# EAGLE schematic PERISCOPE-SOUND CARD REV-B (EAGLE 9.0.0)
This Set of Many Schematics Is what comprises the Revision-B PCB, of my eden project "PERISCOPE". (OBJECT BOARD ONLY)

## Sheet 1 of 3: SOUND
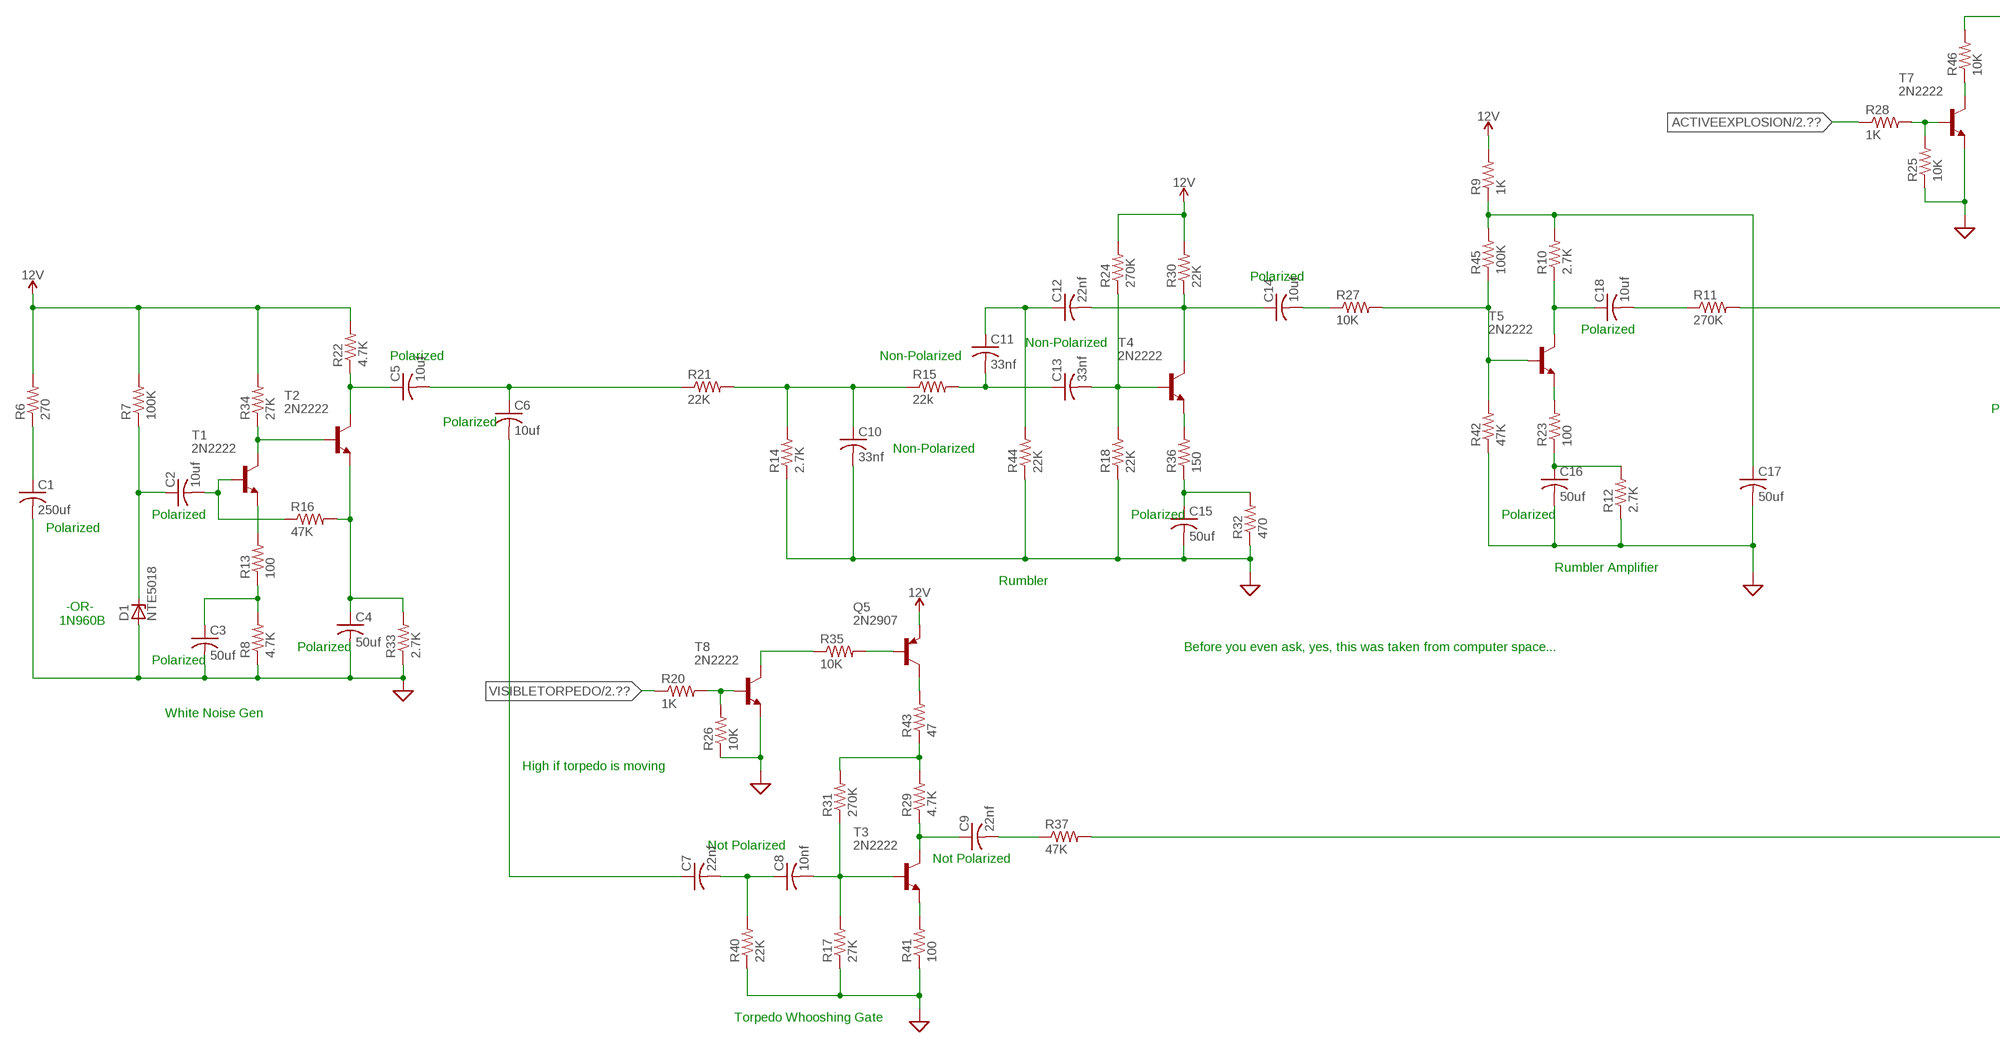
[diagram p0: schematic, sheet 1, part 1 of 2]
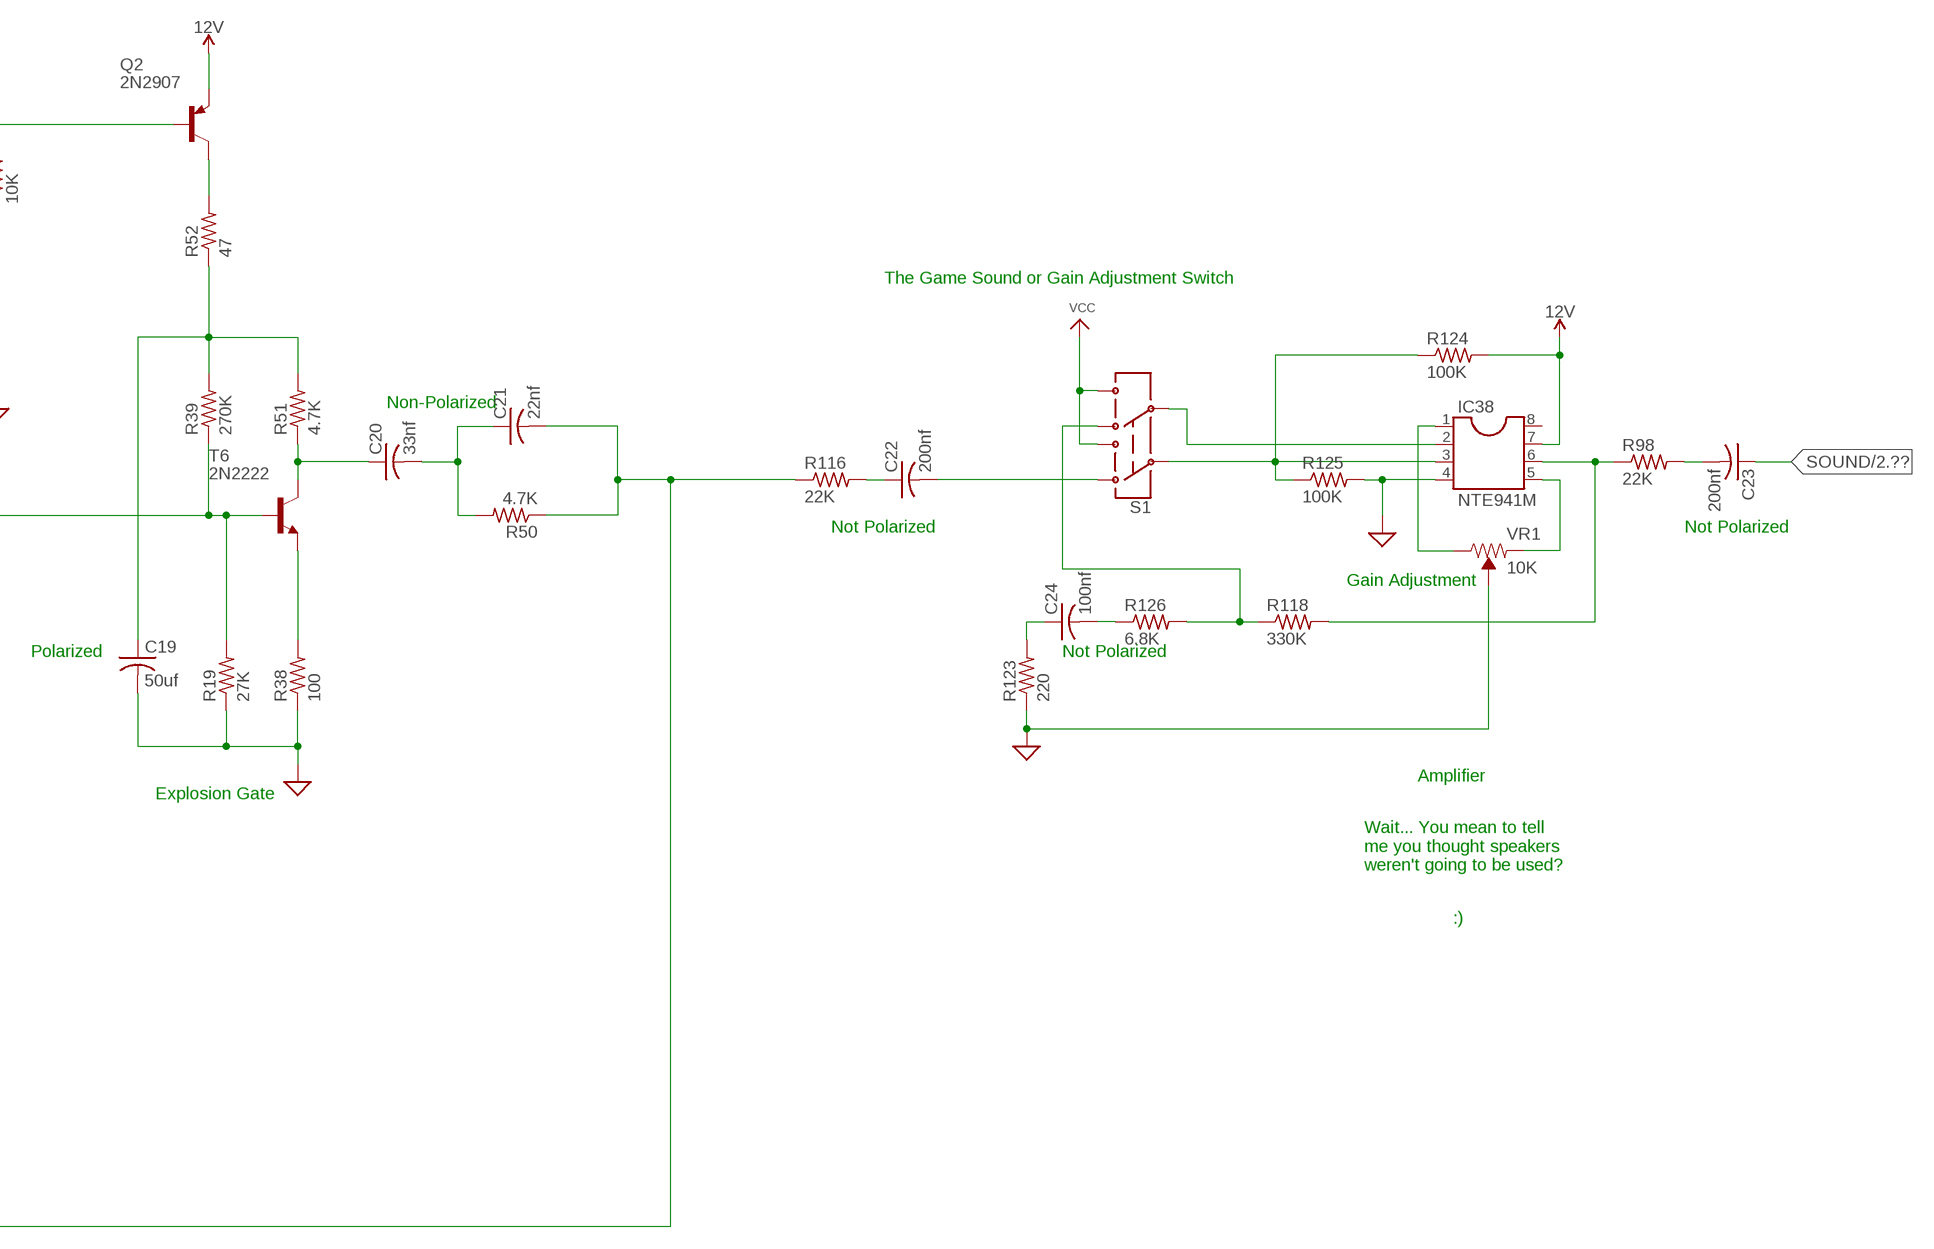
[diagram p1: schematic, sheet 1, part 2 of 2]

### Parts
C1  250uf  C-US025-050X050  [C025-050X050]
C2  10uf  C-US025-050X050  [C025-050X050]
C3  50uf  C-US025-050X050  [C025-050X050]
C4  50uf  C-US025-050X050  [C025-050X050]
C5  10uf  C-US025-050X050  [C025-050X050]
C6  10uf  C-US025-050X050  [C025-050X050]
C7  22nf  C-US025-050X050  [C025-050X050]
C8  10nf  C-US025-050X050  [C025-050X050]
C9  22nf  C-US025-050X050  [C025-050X050]
C10  33nf  C-US025-050X050  [C025-050X050]
C11  33nf  C-US025-050X050  [C025-050X050]
C12  22nf  C-US025-050X050  [C025-050X050]
C13  33nf  C-US025-050X050  [C025-050X050]
C14  10uf  C-US025-050X050  [C025-050X050]
C15  50uf  C-US025-050X050  [C025-050X050]
C16  50uf  C-US025-050X050  [C025-050X050]
C17  50uf  C-US025-050X050  [C025-050X050]
C18  10uf  C-US025-050X050  [C025-050X050]
C19  50uf  C-US025-050X050  [C025-050X050]
C20  33nf  C-US025-050X050  [C025-050X050]
C21  22nf  C-US025-050X050  [C025-050X050]
C22  200nf  C-US050-025X075  [C050-025X075]
C23  200nf  C-US050-025X075  [C050-025X075]
C24  100nf  C-US050-025X075  [C050-025X075]
D1  NTE5018  1N4728  [DO41Z10]
IC38  NTE941M  DIL8S  [SOCKET-08]
Q2  2N2907  [TO92-EBC-OVAL]
Q5  2N2907  [TO92-EBC-OVAL]
R6  270  R-US_0207/10  [0207/10]
R7  100K  R-US_0207/10  [0207/10]
R8  4.7K  R-US_0207/10  [0207/10]
R9  1K  R-US_0207/10  [0207/10]
R10  2.7K  R-US_0207/10  [0207/10]
R11  270K  R-US_0207/10  [0207/10]
R12  2.7K  R-US_0207/10  [0207/10]
R13  100  R-US_0207/10  [0207/10]
R14  2.7K  R-US_0207/10  [0207/10]
R15  22k  R-US_0207/10  [0207/10]
R16  47K  R-US_0207/10  [0207/10]
R17  27K  R-US_0207/10  [0207/10]
R18  22K  R-US_0207/10  [0207/10]
R19  27K  R-US_0207/10  [0207/10]
R20  1K  R-US_0207/10  [0207/10]
R21  22K  R-US_0207/10  [0207/10]
R22  4.7K  R-US_0207/10  [0207/10]
R23  100  R-US_0207/10  [0207/10]
R24  270K  R-US_0207/10  [0207/10]
R25  10K  R-US_0207/10  [0207/10]
R26  10K  R-US_0207/10  [0207/10]
R27  10K  R-US_0207/10  [0207/10]
R28  1K  R-US_0207/10  [0207/10]
R29  4.7K  R-US_0207/10  [0207/10]
R30  22K  R-US_0207/10  [0207/10]
R31  270K  R-US_0207/10  [0207/10]
R32  470  R-US_0207/10  [0207/10]
R33  2.7K  R-US_0207/10  [0207/10]
R34  27K  R-US_0207/10  [0207/10]
R35  10K  R-US_0207/10  [0207/10]
R36  150  R-US_0207/10  [0207/10]
R37  47K  R-US_0207/10  [0207/10]
R38  100  R-US_0207/10  [0207/10]
R39  270K  R-US_0207/10  [0207/10]
R40  22K  R-US_0207/10  [0207/10]
R41  100  R-US_0207/10  [0207/10]
R42  47K  R-US_0207/10  [0207/10]
R43  47  R-US_0207/10  [0207/10]
R44  22K  R-US_0207/10  [0207/10]
R45  100K  R-US_0207/10  [0207/10]
R46  10K  R-US_0207/10  [0207/10]
R50  4.7K  R-US_0207/10  [0207/10]
R51  4.7K  R-US_0207/10  [0207/10]
R52  47  R-US_0207/10  [0207/10]
R98  22K  R-US_0207/10  [0207/10]
R116  22K  R-US_0207/10  [0207/10]
R118  330K  R-US_0207/10  [0207/10]
R123  220  R-US_0207/10  [0207/10]
R124  100K  R-US_0207/10  [0207/10]
R125  100K  R-US_0207/10  [0207/10]
R126  6.8K  R-US_0207/10  [0207/10]
S1  SWITCH-DPDTPTH1  [MS]
T1  2N2222  [TO92-EBC-OVAL]
T2  2N2222  [TO92-EBC-OVAL]
T3  2N2222  [TO92-EBC-OVAL]
T4  2N2222  [TO92-EBC-OVAL]
T5  2N2222  [TO92-EBC-OVAL]
T6  2N2222  [TO92-EBC-OVAL]
T7  2N2222  [TO92-EBC-OVAL]
T8  2N2222  [TO92-EBC-OVAL]
VR1  10K  TRIMPOT-PTH-10MM-KNOB-1/2W-10%  [TRIMPOT-PTH-3386U]

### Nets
12V: IC38.7 Q2.E Q5.E R6.2 R7.2 R9.2 R22.2 R24.2 R30.2 R34.2 R124.2 ; also sheet 2
ACTIVEEXPLOSION: R28.1 ; also sheet 2,3
GND: C1.2 C3.2 C4.2 C10.2 C15.2 C16.2 C17.2 C19.2 D1.A IC38.4 R8.1 R12.1 R14.1 R17.1 R18.1 R19.1 R25.1 R26.1 R32.1 R33.1 R38.1 R40.1 R41.1 R42.1 R44.1 R123.1 R125.2 T7.E T8.E VR1.2(WIPER) ; supply symbol labelled SUP ; also sheet 2
N$1: C21.2 R37.2 R50.1 R116.1
N$3: R13.2 T1.E
N$4: C1.1 R6.1
N$5: C2.1 D1.C R7.1
N$6: C3.1 R8.2 R13.1
N$7: C9.2 R37.1
N$8: C2.2 R16.1 T1.B
N$10: R34.1 T1.C T2.B
N$11: C4.1 R16.2 R33.2 T2.E
N$12: C10.1 R14.2 R15.1 R21.2
N$13: C5.1 R22.1 T2.C
N$14: C5.2 C6.1 R21.1
N$15: C6.2 C7.1
N$16: C7.2 C8.1 R40.2
N$17: C11.2 C13.1 R15.2
N$18: C8.2 R17.2 R31.1 T3.B
N$19: R29.2 R31.2 R43.1
N$20: C9.1 R29.1 T3.C
N$21: R41.2 T3.E
N$22: Q5.C R43.2
N$23: Q5.B R35.2
N$24: R35.1 T8.C
N$25: R20.2 R26.2 T8.B
N$26: C11.1 C12.1 R44.2
N$27: C12.2 C14.1 R30.1 T4.C
N$28: C13.2 R18.2 R24.1 T4.B
N$29: R36.2 T4.E
N$30: C15.1 R32.2 R36.1
N$31: R27.2 R42.2 R45.1 T5.B
N$32: C14.2 R27.1
N$33: Q2.B R46.2
N$34: C16.1 R12.2 R23.1
N$35: R23.2 T5.E
N$36: C18.1 R10.1 T5.C
N$37: C17.1 R9.1 R10.2 R45.2
N$38: C18.2 R11.1
N$39: R11.2 R19.2 R39.1 T6.B
N$40: R25.2 R28.2 T7.B
N$42: R46.1 T7.C
N$43: Q2.C R52.2
N$44: C20.2 C21.1 R50.2
N$45: C19.1 R39.2 R51.2 R52.1
N$46: C20.1 R51.1 T6.C
N$47: R38.2 T6.E
N$117: IC38.2 S1.5
N$118: IC38.5 VR1.1(CCW)
N$169: R118.1 R126.2 S1.4
N$178: C22.1 R116.2
N$180: C22.2 S1.1
N$181: C23.2 R98.2
N$182: IC38.1 VR1.3(CW)
N$184: IC38.6 R98.1 R118.2
N$188: IC38.3 R124.1 R125.1 S1.2
N$193: C24.1 R123.2
N$194: C24.2 R126.1
SOUND: C23.1 ; also sheet 2,3
VCC: S1.3 S1.6
VISIBLETORPEDO: R20.1 ; also sheet 2,3
Unconnected: IC38.8

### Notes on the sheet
- The Game Sound or Gain Adjustment Switch
- Non-Polarized
- Polarized
- Not Polarized | Not Polarized
- Polarized
- Non-Polarized
- Polarized | Non-Polarized | Gain Adjustment
- Polarized | Not Polarized
- Polarized
- Non-Polarized
- Amplifier
- Polarized | Polarized | Polarized | Explosion Gate
- Polarized
- Rumbler Amplifier
- Wait... You mean to tell
  me you thought speakers
  weren't going to be used?
- Rumbler
- :)
- -OR-
  1N960B
- Polarized | Before you even ask, yes, this was taken from computer space...
- Polarized
- White Noise Gen
- High if torpedo is moving
- Not Polarized
- Not Polarized
- Torpedo Whooshing Gate

## Sheet 2 of 3: Signal Connectors
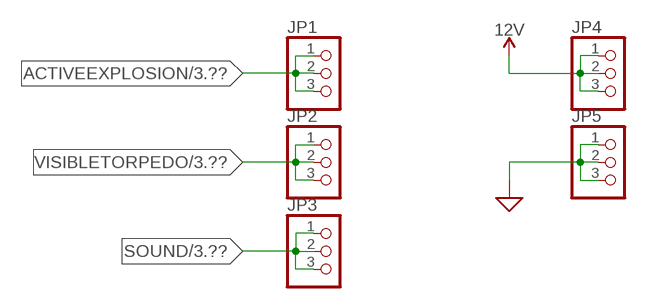
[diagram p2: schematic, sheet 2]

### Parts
JP1  PINHD-1X3  [1X03]
JP2  PINHD-1X3  [1X03]
JP3  PINHD-1X3  [1X03]
JP4  PINHD-1X3  [1X03]
JP5  PINHD-1X3  [1X03]

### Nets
12V: JP4.1 JP4.2 JP4.3 ; also sheet 1
ACTIVEEXPLOSION: JP1.1 JP1.2 JP1.3 ; also sheet 1,3
GND: JP5.1 JP5.2 JP5.3 ; supply symbol labelled SUP ; also sheet 1
SOUND: JP3.1 JP3.2 JP3.3 ; also sheet 1,3
VISIBLETORPEDO: JP2.1 JP2.2 JP2.3 ; also sheet 1,3

## Sheet 3 of 3: Alt. Sound
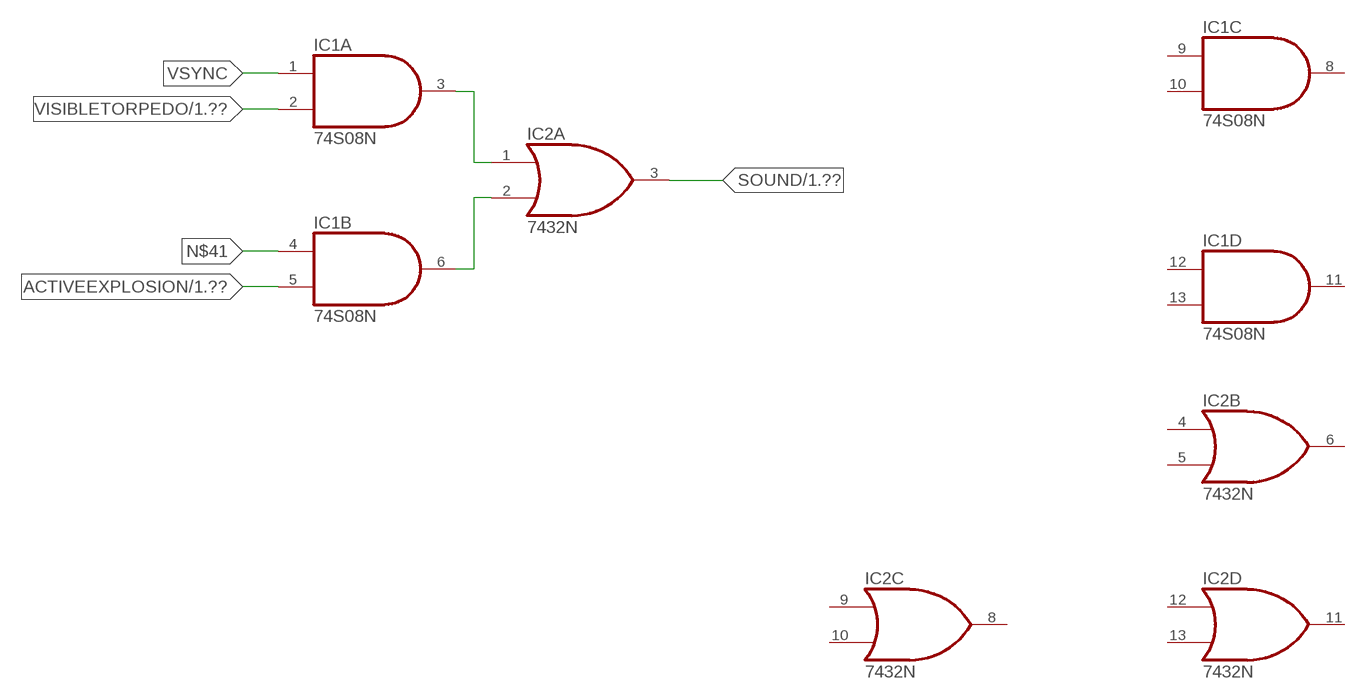
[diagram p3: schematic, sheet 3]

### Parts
IC1  74S08N  [DIL14]
IC2  7432N  [DIL14]

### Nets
ACTIVEEXPLOSION: IC1.5(B:I1) ; also sheet 1,2
N$2: IC1.3(A:O) IC2.1(A:I0)
N$9: IC1.6(B:O) IC2.2(A:I1)
N$41: IC1.4(B:I0)
SOUND: IC2.3(A:O) ; also sheet 1,2
VISIBLETORPEDO: IC1.2(A:I1) ; also sheet 1,2
VSYNC: IC1.1(A:I0)
Unconnected: IC1.8(C:O) IC1.9(C:I0) IC1.10(C:I1) IC1.11(D:O) IC1.12(D:I0) IC1.13(D:I1) IC2.4(B:I0) IC2.5(B:I1) IC2.6(B:O) IC2.8(C:O) IC2.9(C:I0) IC2.10(C:I1) IC2.11(D:O) IC2.12(D:I0) IC2.13(D:I1)

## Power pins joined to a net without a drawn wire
GND: IC1.7(P:GND) IC2.7(P:GND)
VCC: IC1.14(P:VCC) IC2.14(P:VCC)

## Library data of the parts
C1-C24 = adafruit:C-US: CAPACITOR, American symbol
D1 = diode:1N4728: Z DIODE
IC1 = 74xx-us:74*08: Quad 2-input AND gate
IC2 = 74xx-us:74*32: Quad 2-input OR gate
IC38 = ic-package:DIL8: Dual In Line / Socket
JP1-JP5 = adafruit:PINHD-1X3: PIN HEADER
Q2 Q5 = adafruit:2N2907*: PNP Transistor Big Oval pads
R6-R46 R50-R52 R98 R116 R118 R123-R126 = adafruit:R-US_: RESISTOR, American symbol
S1 = SparkFun-Retired:SWITCH-DPDT: DPDT Version of the COM-00597; SF_SKU: COM-11139
T1-T8 = adafruit:2N2222: NPN TRANSISTOR Big oval pads
VR1 = SparkFun-Resistors:TRIMPOT: Trimming Potentiometer (Trimpot) Three-terminal potentiometers, with an adjustable wiper and two adjustable resistors. A pot can be used to create a configurable voltage divider, or as a variable resistor. "Trimpots" are a subset of potentiometers, usually intended for "set-and-forget"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; PROD_ID: RES-09730; SF_SKU: COM-09806; VALUE: 10k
